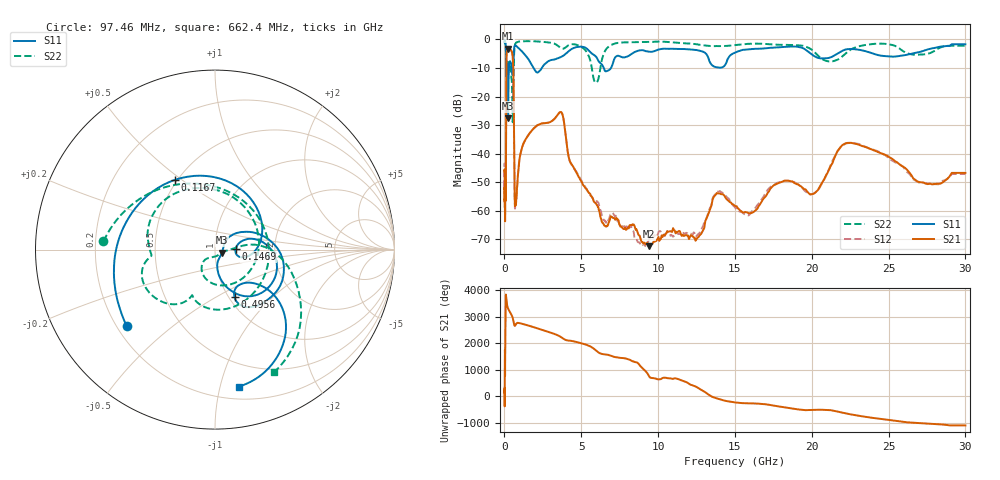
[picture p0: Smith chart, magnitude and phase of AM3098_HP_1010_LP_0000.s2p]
! Date/Time: Thu, Feb 28, 2019 8:41 AM
! Network Analyzer: Agilent Technologies E8364B Rev: A.07.50.67
! Sweep from 0.010 to 30.000 GHz, 1601 Points, Sweep Type: LOG
! Power Supply: 5.022 V, 0.002 A
# Hz S DB R 50
!freq MagS11 AngS11 MagS21 AngS21 MagS12 AngS12 MagS22 AngS22
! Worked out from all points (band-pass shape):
!   1601 points, 10 MHz to 30 GHz, reference 50 ohm
!   highest |S21| = -3.28 dB at 241.1 MHz (marker M1); lowest = -72.4 dB at 9.396 GHz (marker M2)
!   |S21| within 3 dB of the highest: 133 MHz to 538.4 MHz (405.4 MHz wide, 121 % of centre)
!   lowest |S11| = -27.5 dB at 238.7 MHz (marker M3), VSWR 1.09, Z = 54 - j1.77 ohm
!   |S11| at or under -10 dB: 199.7 MHz to 293.3 MHz (93.64 MHz wide, 38 % of centre); 1.888 GHz to 2.428 GHz (539.6 MHz wide, 25 % of centre); 6.466 GHz to 6.934 GHz (467.9 MHz wide, 6.98 % of centre)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
!   |S22| runs from -29.0 to -0.5 dB; largest |S21 - S12| = 0.0091
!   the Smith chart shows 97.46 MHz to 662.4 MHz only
!   S11 on the Smith chart (normalised r, x): 97.46 MHz: 0.24, -0.35; 116.7 MHz: 0.49, +0.47; 146.9 MHz: 1.26, +0.01; 495.6 MHz: 1.06, -0.61; 662.4 MHz: 0.30, -1.14
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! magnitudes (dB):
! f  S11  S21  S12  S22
! 10 MHz  -0.4  -46.2  -45.8  -0.5
! 38.04 MHz  -0.4  -60.2  -61.4  -0.7
! 97.46 MHz  -3.7  -46.5  -49.2  -4.1
! 116.7 MHz  -7.0  -17.8  -17.8  -10.4
! 144.7 MHz  -18.8  -4.7  -4.6  -10.8
! 146.9 MHz  -18.8  -4.5  -4.5  -10.5
! 191.5 MHz  -9.0  -3.8  -3.8  -7.2
! 238.7 MHz  -27.5  -3.3  -3.2  -9.0
! 241.1 MHz  -27.4  -3.3  -3.2  -9.0
! 306.5 MHz  -8.9  -3.5  -3.5  -8.0
! 495.6 MHz  -10.9  -4.6  -4.5  -17.2
! 550.5 MHz  -11.2  -7.2  -7.2  -27.4
! 593.4 MHz  -5.8  -16.0  -15.9  -12.0
! 662.4 MHz  -2.2  -54.2  -55.3  -2.4
! 2.084 GHz  -11.5  -30.3  -30.3  -0.7
! 3.686 GHz  -6.1  -25.4  -25.4  -3.1
! 5.959 GHz  -6.0  -57.5  -56.8  -15.1
! 7.926 GHz  -6.1  -66.7  -65.6  -1.0
! 9.396 GHz  -4.3  -72.4  -70.1  -0.9
! 20 GHz  -5.3  -54.2  -54.1  -3.6
! 22.56 GHz  -3.3  -36.2  -36.2  -3.5
! 30 GHz  -1.7  -46.7  -47.1  -2.2
